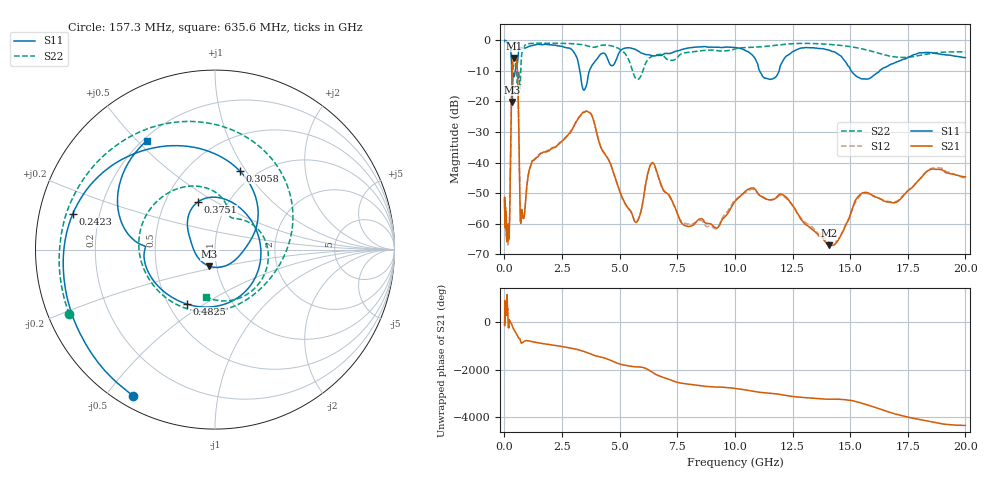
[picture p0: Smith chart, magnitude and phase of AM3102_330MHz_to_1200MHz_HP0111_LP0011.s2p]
! Date/Time: Tue, Sep 11, 2018 5:15 PM
! Network Analyzer: Agilent Technologies E8362B Rev: A.07.50.63
! Sweep from 0.010 to 20.000 GHz, 1601 Points, Sweep Type: LOG
! Power Supply: 4.949 V, 0.001 A
# Hz S DB R 50
!freq MagS11 AngS11 MagS21 AngS21 MagS12 AngS12 MagS22 AngS22
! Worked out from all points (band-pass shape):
!   1601 points, 10 MHz to 20 GHz, reference 50 ohm
!   highest |S21| = -5.75 dB at 434.6 MHz (marker M1); lowest = -67.2 dB at 14.07 GHz (marker M2)
!   |S21| within 3 dB of the highest: 347.7 MHz to 556.3 MHz (208.6 MHz wide, 46.1 % of centre)
!   lowest |S11| = -20.2 dB at 341.1 MHz (marker M3), VSWR 1.22, Z = 46.2 - j8.65 ohm
!   |S11| at or under -10 dB: 3.276 GHz to 3.685 GHz (409.6 MHz wide, 11.8 % of centre); 11.07 GHz to 11.92 GHz (846.1 MHz wide, 7.36 % of centre); 15.04 GHz to 16.28 GHz (1.233 GHz wide, 7.87 % of centre)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
!   |S22| runs from -15.8 to -0.2 dB; largest |S21 - S12| = 0.0075
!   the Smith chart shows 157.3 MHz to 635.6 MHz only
!   S11 on the Smith chart (normalised r, x): 157.3 MHz: 0.05, -0.59; 242.3 MHz: 0.10, +0.12; 305.8 MHz: 0.84, +0.94; 375.1 MHz: 0.73, +0.42; 482.5 MHz: 0.62, -0.42; 635.6 MHz: 0.21, +0.53
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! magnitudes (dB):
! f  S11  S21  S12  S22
! 10 MHz  0.0  -52.6  -54.0  -0.2
! 35.55 MHz  0.0  -59.0  -58.6  -0.4
! 126.4 MHz  -0.4  -64.8  -63.1  -0.9
! 157.3 MHz  -0.6  -63.5  -66.5  -1.0
! 242.3 MHz  -1.8  -51.6  -51.9  -1.9
! 305.8 MHz  -6.7  -20.4  -20.4  -4.5
! 341.1 MHz  -20.2  -9.7  -9.8  -8.6
! 375.1 MHz  -11.0  -6.8  -6.9  -9.3
! 434.6 MHz  -11.6  -5.7  -5.8  -7.5
! 447.2 MHz  -11.0  -5.8  -5.8  -7.4
! 482.5 MHz  -9.3  -6.0  -6.1  -7.6
! 567.1 MHz  -7.4  -10.2  -10.4  -13.8
! 635.6 MHz  -2.9  -33.5  -33.6  -11.4
! 709 MHz  -2.4  -59.9  -60.2  -10.1
! 1.59 GHz  -1.4  -37.0  -37.0  -0.9
! 3.651 GHz  -10.9  -23.5  -23.2  -1.9
! 5.652 GHz  -2.9  -59.3  -59.1  -11.9
! 6.457 GHz  -5.1  -40.1  -40.4  -5.0
! 7.882 GHz  -2.7  -60.8  -60.0  -4.0
! 10.73 GHz  -4.6  -48.3  -48.8  -2.3
! 14.07 GHz  -3.1  -67.2  -66.1  -1.3
! 20 GHz  -5.6  -44.7  -45.2  -3.7
